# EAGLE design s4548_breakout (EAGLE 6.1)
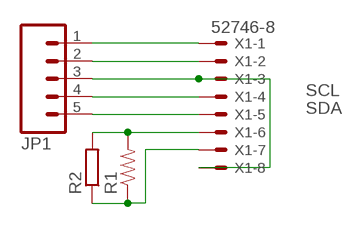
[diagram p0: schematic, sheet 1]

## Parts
JP1  M05PTH_LONGPADS  [1X05_LONGPADS]
R1  RESISTOR0603-RES  [0603-RES]
R2  R-EU_0204/2V  [0204V]
X1  52746-8  [52746-8]

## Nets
GND: JP1.2 X1.2
N$6: R1.2 R2.2 X1.6
N$7: R1.1 R2.1 X1.7
SCL: JP1.4 X1.4
SDA: JP1.5 X1.5
VDD: JP1.3 X1.3 X1.8
VLCD: JP1.1 X1.1

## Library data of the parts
JP1 = SparkFun:M05: Header 5 Standard 5-pin 0.1" header. Use with straight break away headers (SKU : PRT-00116), right angle break away headers (PRT-00553), swiss pins (PRT-00743), machine pins (PRT-00117), and female headers (PRT-00115). Molex polarized connector foot print use with SKU : PRT-08230 with associated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
R1 = SparkFun:RESISTOR: Resistor
R2 = rcl:R-EU_: RESISTOR, European symbol
X1 = con-molex:52746-8: FPC Connector ZIF for SMT 0.5mm Source: http://www.farnell.com/datasheets/73044.pdf [DWG. NO. (Sheet 1 OF 2) SD-52746-**17]; OC_FARNELL: unknown; OC_NEWARK: unknown

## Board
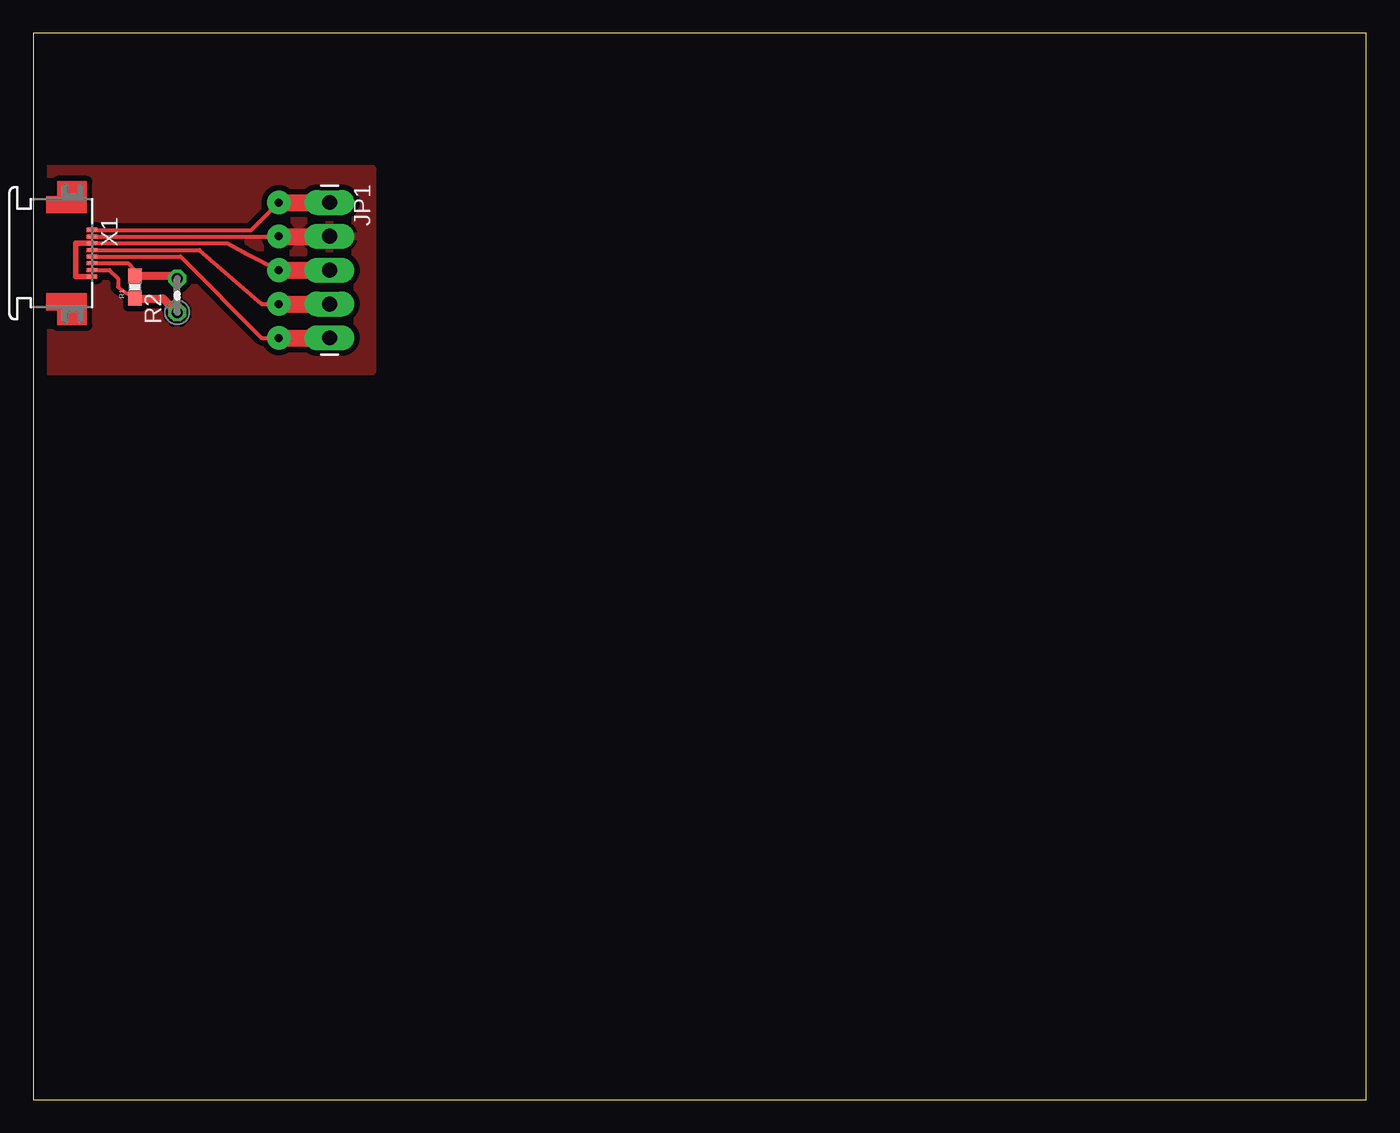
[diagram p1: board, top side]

Size 100 x 80 mm. Coordinates in mm from the lower left corner, seen from the top.
Outline: 0,0 100,0 100,80 0,80 0,0
Copper layers (1*16): Top 0.035mm / dielectric 1.5mm / Bottom 0.035mm
Design rules: minimum track width 10mil, minimum drill 24mil, track to track 8mil, track to pad 8mil, pad to pad 8mil, via to via 8mil, smd to smd 8mil, copper to edge 40mil, drill to drill 8mil, minimum pad ring 10mil, minimum via ring 8mil, stop-mask expansion 4mil, vias tented up to drill 0mil, thermal gap 10mil

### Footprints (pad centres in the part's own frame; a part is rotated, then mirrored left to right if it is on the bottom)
1X05_LONGPADS = drill 1.118 pad 1.88 long: 1 0,0; 2 2.54,0; 3 5.08,0; 4 7.62,0; 5 10.16,0
0603-RES = smd 1.1 x 1: 1 -0.85,0; 2 0.85,0
0204V = drill 0.813 octagon: 1 -1.27,0; 2 1.27,0
52746-8 = smd 0.3 x 0.8: 1 -1.75,0.6; 2 -1.25,0.6; 3 -0.75,0.6; 4 -0.25,0.6; 5 0.25,0.6; 6 0.75,0.6; 7 1.25,0.6; 8 1.75,0.6

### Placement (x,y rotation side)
JP1  22.23,67.31 270 top
R1  7.62,60.96 90 top
R2  10.79,60.33 90 top
X1  3.81,63.5 270 top

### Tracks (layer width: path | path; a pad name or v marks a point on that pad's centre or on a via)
GND
  Top 0.305: X1.2 18.39,64.75 18.41,64.77
  Top 1.27: 18.39,64.75 22.2,64.75 JP1.2
  pour Top (isolate 0.406): -1.27,69.85 25.4,69.85 25.4,54.61 -1.27,54.61
N$6
  Top 0.305: R1.2 7.83,61.81 7.62,62.23 7.1,62.75 X1.6
  Top 0.61: R1.2 10.58,61.81 R2.2
N$7
  Top 0.305: R1.1 6.35,60.96 6.35,61.59 5.7,62.25 X1.7
  Top 0.61: R1.1 9.74,60.11 R2.1
N$8  (via drill 0.6 pad 1.78)
  other vias: 18.41,67.31
N$9  (via drill 0.6 pad 1.78)
  other vias: 18.41,64.77
N$10  (via drill 0.6 pad 1.78)
  other vias: 18.41,62.23
SCL  (via drill 0.6 pad 1.78)
  Top 0.305: X1.4 12.45,63.75 17.14,59.69 v18.41,59.69
  Top 1.27: v18.41,59.69 JP1.4
SDA  (via drill 0.6 pad 1.78)
  Top 0.305: X1.5 11.04,63.25 17.14,57.15 v18.41,57.15
  Top 1.27: v18.41,57.15 JP1.5
VDD
  Top 0.305: 18.41,62.23 15.88,63.5 14.49,64.25 X1.3
  Top 0.406: X1.8 3.17,61.75 3.17,64.25 X1.3
  Top 1.27: 18.41,62.23 JP1.3
VLCD
  Top 0.305: X1.1 16.36,65.25 18.41,67.31
  Top 1.27: 18.41,67.31 JP1.1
